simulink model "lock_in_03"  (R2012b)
settings: Solver=FixedStepDiscrete  StartTime=0.0  StopTime=0.5  FixedStep=1e-5  MaxStep=1/(100e3)  RelTol=1e-3
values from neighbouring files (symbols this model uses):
  a = [m1, c1, k1]    [feder_masse_1.m]    (also in feder_masse_11.m = [m1, c1(1), k1]; feder_masse_12.m = [1/(w01^2), 2*zeta(p)/w01, 1]; suspension_1.m = 1.7; suspension_2.m = 1.7)
  A = 1000    [lock_in01.m]    (also in lock_in011.m; lock_in02.m; lock_in03.m; feder_masse_1.m = [0 1 0 0;-(k1+k2)/m1,-(c1+c2)/m1, k2/m1,c2/m1)
  ampl_ref = 1    [lock_in01.m]    (also in lock_in011.m; lock_in02.m; lock_in03.m)
  ampl_sig = Usig*sqrt(2)    [lock_in01.m]    (also in lock_in011.m; lock_in02.m; lock_in03.m)
  b = 1    [feder_masse_1.m]    (also in feder_masse_11.m; feder_masse_12.m)
  fsig = 10e3    (= 10000)    [lock_in01.m]    (also in lock_in011.m; lock_in02.m; lock_in03.m; diff_filter_1.m = 1)
  L = 0.001    [boost_up1.m]    (also in buck_boost1.m; buck_boost2.m; buck_down1.m; buck_down2.m)
  phase_ref = 0    [lock_in01.m]    (also in lock_in011.m; lock_in02.m; lock_in03.m)
  phase_sig = 0    [lock_in01.m]    (also in lock_in011.m; lock_in02.m; lock_in03.m)
  Ts = 1e-5    (= 1e-05)    [lock_in01.m]    (also in lock_in011.m; lock_in02.m; lock_in03.m)
  v_rausch = (rausch_effektiv)^2*fs    (= 2.5e-12)    [lock_in01.m]    (also in lock_in011.m; lock_in02.m; lock_in03.m)
undefined symbols (not defined in the file or in its folder): dBW, Fs, get, Hertz, sided, Two
libraries: dspsigops x2, dspsnks4 x2, dspstat3 x1

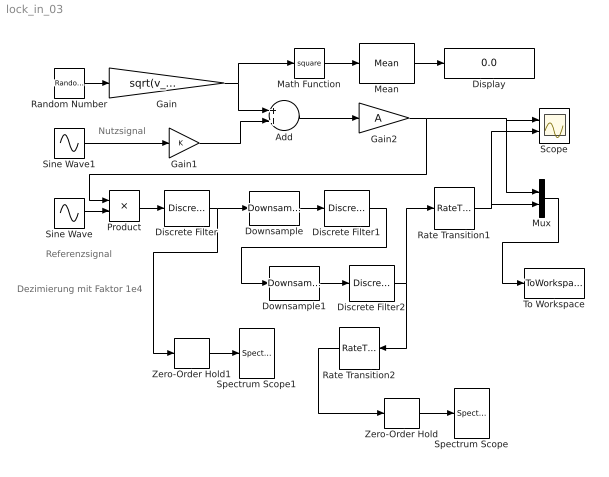
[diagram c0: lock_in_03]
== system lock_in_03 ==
  note: Dezimierung mit Faktor 1e4
  note: Referenzsignal
  note: Nutzsignal
  Add : Sum
  Discrete Filter : DiscreteFilter  Numerator=[b]  Denominator=[a]  SampleTime=Ts
  Discrete Filter1 : DiscreteFilter  Numerator=[b]  Denominator=[a]  SampleTime=Ts*100
  Discrete Filter2 : DiscreteFilter  Numerator=[b]  Denominator=[a]  SampleTime=Ts*10000
  Display : Display
  Downsample : dspsigops/Downsample  N=L  phase=0  RateOptions=Allow multirate processing  smode=Force single rate  fmode=Maintain input frame size  ic=0
  Downsample1 : dspsigops/Downsample  N=L  phase=0  RateOptions=Allow multirate processing  smode=Force single rate  fmode=Maintain input frame size  ic=0
  Gain : Gain  Gain=sqrt(v_rausch)
  Gain1 : Gain
  Gain2 : Gain  Gain=A
  Math Function : Math  Operator=square
  Mean : dspstat3/Mean  run=on  reset_popup=None  InputProcessing=Columns as channels (frame based)  directionMode=Each column  dimension=1  treatSBRowAsCol=on  roiEnable=off  roiType=Rectangles  roiPortion=Entire ROI  roiOutput=Individual statistics for each ROI  roiFlag=off  outputDataTypeStr=Inherit: Same as accumulator  outputLastDataTypeStr=Inherit: Same as accumulator  outputMin=[]  outputMax=[]  roundingMode=Floor  overflowMode=off
  Mux : Mux  Inputs=2
  Product : Product
  Random Number : RandomNumber  SampleTime=Ts
  Rate Transition1 : RateTransition  OutPortSampleTime=Ts
  Rate Transition2 : RateTransition  OutPortSampleTime=1/50
  Scope : Scope  NumInputPorts=2
  Sine Wave : Sin  Amplitude=ampl_ref  Frequency=2*pi*fsig  Phase=phase_ref  SampleTime=Ts
  Sine Wave1 : Sin  Amplitude=ampl_sig  Frequency=2*pi*fsig  Phase=phase_sig  SampleTime=Ts
  Spectrum Scope : dspsnks4/Spectrum Scope  ScopeProperties=on  Domain=Frequency  HorizSpan=1  UseBuffer=on  BufferSize=256  Overlap=0  TreatMby1Signals=One channel  inpFftLenInherit=on  FFTlength=256  numAvg=1  DisplayProperties=off  AxisGrid=on  Memory=off  FrameNumber=on  AxisLegend=off  AxisZoom=off  OpenScopeAtSimStart=on  OpenScopeImmediately=off  FigPos=get(0,'defaultfigureposition')  AxisProperties=off  XUnits=Hertz  XRange=Two-sided ((-Fs/2...Fs/2])  XDisplay=0  InheritXIncr=on  XIncr=0.02  XLabel=Samples  XLimit=User-defined  YUnits=dBW/Hertz  XMax=25  XMin=-25  YLabel=Magnitude-squared, dB  LineProperties=off  wintypeSpecScope=Hamming  RsSpecScope=50  betaSpecScope=5  winsampSpecScope=Periodic  XAxisParamsVer=6.9  isFrameUpgraded=on
  Spectrum Scope1 : dspsnks4/Spectrum Scope  ScopeProperties=on  Domain=Frequency  HorizSpan=1  UseBuffer=on  BufferSize=256  Overlap=0  TreatMby1Signals=One channel  inpFftLenInherit=on  FFTlength=256  numAvg=10  DisplayProperties=off  AxisGrid=on  Memory=off  FrameNumber=on  AxisLegend=off  AxisZoom=off  OpenScopeAtSimStart=on  OpenScopeImmediately=off  FigPos=get(0,'defaultfigureposition')  AxisProperties=off  XUnits=Hertz  XRange=Two-sided ((-Fs/2...Fs/2])  XDisplay=0  InheritXIncr=on  XIncr=0.02  XLabel=Samples  XLimit=User-defined  YUnits=dBW/Hertz  XMax=1000  XMin=-1000  YLabel=Magnitude-squared, dB  LineProperties=off  wintypeSpecScope=Hamming  RsSpecScope=50  betaSpecScope=5  winsampSpecScope=Periodic  XAxisParamsVer=6.9  isFrameUpgraded=on
  To Workspace : ToWorkspace  VariableName=y  SampleTime=-1  SaveFormat=Structure With Time
  Zero-Order Hold : ZeroOrderHold  SampleTime=1/50
  Zero-Order Hold1 : ZeroOrderHold  SampleTime=1/2000
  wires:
  Sine Wave/1 -> Product/2
  Random Number/1 -> Gain/1
  Sine Wave1/1 -> Gain1/1
  Gain1/1 -> Add/2
  Gain/1 -> Add/1, Math Function/1
  Add/1 -> Gain2/1
  Product/1 -> Discrete Filter/1
  Math Function/1 -> Mean/1
  Mean/1 -> Display/1
  Mux/1 -> To Workspace/1
  Downsample/1 -> Discrete Filter1/1
  Gain2/1 -> Product/1, Mux/1, Scope/1
  Rate Transition1/1 -> Mux/2, Scope/2
  Zero-Order Hold/1 -> Spectrum Scope/1
  Zero-Order Hold1/1 -> Spectrum Scope1/1
  Discrete Filter/1 -> Zero-Order Hold1/1, Downsample/1
  Downsample1/1 -> Discrete Filter2/1
  Discrete Filter1/1 -> Downsample1/1
  Discrete Filter2/1 -> Rate Transition2/1, Rate Transition1/1
  Rate Transition2/1 -> Zero-Order Hold/1
